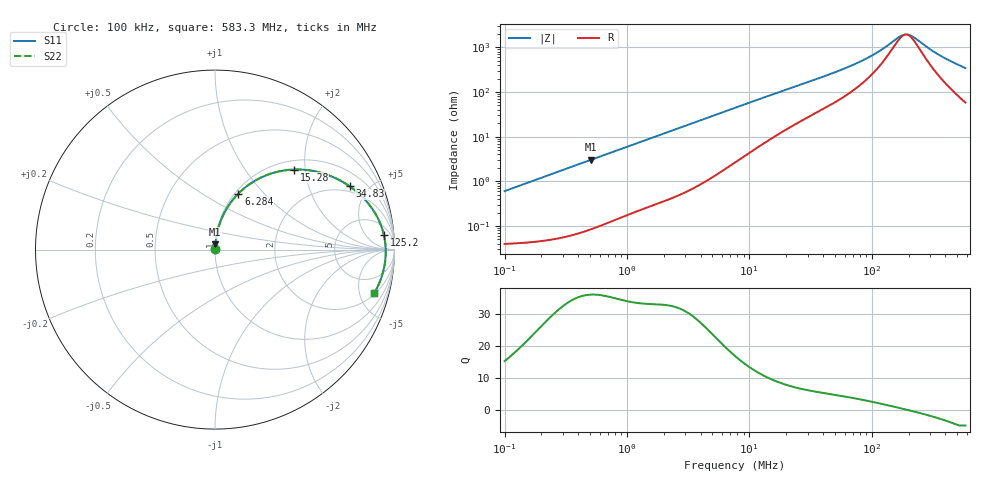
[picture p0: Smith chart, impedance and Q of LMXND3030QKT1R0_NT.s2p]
! LMXND3030QKT1R0_NT  S-PARAMETER MODEL  ( Standard Model )
! Model Generated by TAIYO YUDEN Corporation (https://www.yuden.co.jp/en/)
! Version 1.0
! TAIYO YUDEN Control No. 20250724
! Copyright(c) 2025 TAIYO YUDEN CO.,LTD. All Rights Reserved.
! Product Description (link to TY-COMPAS)
! https://ds.yuden.co.jp/TYCOMPAS/or/detail?pn=LMXND3030QKT1R0NNT&u=M
! Products Name : Inductors
! Characteristics :
!  Inductance : 1.0 [uH] , SRF(min) : 100 [MHz] , DC Resistance(max) : 0.036 [Ohm]
!  Rated Current : Saturation  2100 [m A] , Temp Rise  3000 [m A] (40 [degC])
!  Case Size : 3.0 x 3.0 / 0.118 x 0.118 [mm/inch] , Thickness : 1.5 / 0.059 [mm/inch]
!  (Conditions: Temperature = 25 [degC] , DC Bias Current = 0 [A])
! External Node Assignments :
!  1  o---GGG---o  2
! GND o---------o GND
! Frequency Range : 0.1MHz  -  583.332491MHz  [ 402 STEP ]
# MHz S RI R 50
! Freq[MHz].  S11 Real  S11 Imag  S21 Real  S21 Imag  S12 Real  S12 Imag  S22 Real  S22 Imag
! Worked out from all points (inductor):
!   401 points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, 100 kHz to 583.3 MHz, reference 50 ohm
!   read as one part in series: L = 959 nH near 104.4 kHz
!   highest Q = 36.1 at 508.3 kHz (marker M1), where L = 953 nH
!   self-resonance near 190.5 MHz
!   S11 on the Smith chart (normalised r, x): 100 kHz: 1.00, +0.01; 6.284 MHz: 1.04, +0.73; 15.28 MHz: 1.18, +1.74; 34.83 MHz: 1.68, +3.78; 125.2 MHz: 11, +16; 583.3 MHz: 2.16, -6.80
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0.1  0.000433 0.00603  0.9996 -0.00603  0.9996 -0.00603  0.000433 0.00603
0.427357  0.00137 0.0256  0.9986 -0.0256  0.9986 -0.0256  0.00137 0.0256
0.508287  0.00177 0.0303  0.9982 -0.0303  0.9982 -0.0303  0.00177 0.0303
1.826341  0.0145 0.1054  0.9855 -0.1054  0.9855 -0.1054  0.0145 0.1054
3.734823  0.0521 0.2052  0.9479 -0.2052  0.9479 -0.2052  0.0521 0.2052
6.283838  0.1304 0.3124  0.8696 -0.3124  0.8696 -0.3124  0.1304 0.3124
7.637621  0.179 0.3548  0.821 -0.3548  0.821 -0.3548  0.179 0.3548
11.04103  0.3038 0.4209  0.6962 -0.4209  0.6962 -0.4209  0.3038 0.4209
15.2838  0.4395 0.4461  0.5605 -0.4461  0.5605 -0.4461  0.4395 0.4461
21.62061  0.5857 0.4294  0.4143 -0.4294  0.4143 -0.4294  0.5857 0.4294
32.63992  0.7315 0.3652  0.2685 -0.3652  0.2685 -0.3652  0.7315 0.3652
34.8332  0.7507 0.3524  0.2493 -0.3524  0.2493 -0.3524  0.7507 0.3524
50.35526  0.8399 0.2735  0.1601 -0.2735  0.1601 -0.2735  0.8399 0.2735
72.79412  0.8984 0.1918  0.1016 -0.1918  0.1016 -0.1918  0.8984 0.1918
96.49139  0.9259 0.132  0.0741 -0.132  0.0741 -0.132  0.9259 0.132
125.1601  0.9413 0.0799  0.0587 -0.0799  0.0587 -0.0799  0.9413 0.0799
139.489  0.9454 0.0589  0.0546 -0.0589  0.0546 -0.0589  0.9454 0.0589
177.0528  0.9506 0.0138  0.0494 -0.0138  0.0494 -0.0138  0.9506 0.0138
201.6468  0.9513 -0.0107  0.0487 0.0107  0.0487 0.0107  0.9513 -0.0107
219.9128  0.951 -0.0272  0.049 0.0272  0.049 0.0272  0.951 -0.0272
362.0685  0.9355 -0.128  0.0645 0.128  0.0645 0.128  0.9355 -0.128
583.3325  0.8874 -0.2419  0.1126 0.2419  0.1126 0.2419  0.8874 -0.2419
